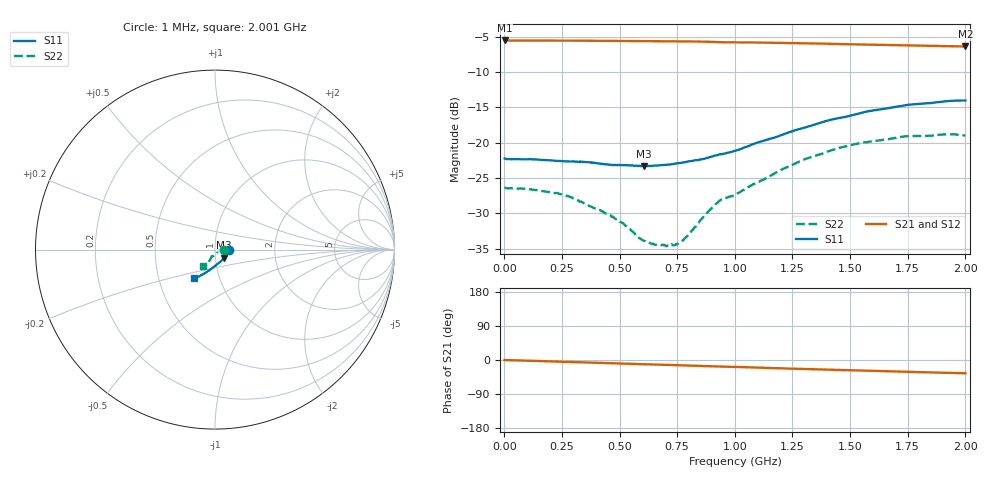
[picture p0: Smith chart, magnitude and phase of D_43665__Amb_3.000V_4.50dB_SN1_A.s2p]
! device id: 43665_
! dir: \\malibu\benchdata\1_engineers\tn_data\43665_75ohm\new\sparar\43665_\amb\3p000v\4p50db
! Serial: 1
! Insertion: A
! Temp: Amb
! VDD: 3.000V
! Attenuation Step: 4.50dB
! IDD: 1.453503e+00mA
! FILE NAME
! DATE 03-27-2009 08:34:29
! CORRECTED  DATA
#  Hz  S  RI  R  75
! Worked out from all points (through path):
!   401 points, 1 MHz to 2.001 GHz, reference 75 ohm
!   highest |S21| = -5.54 dB at 1 MHz (marker M1); lowest = -6.4 dB at 2.001 GHz (marker M2)
!   group delay of S21, straight-line fit = 49.6 ps
!   lowest |S11| = -23.3 dB at 606 MHz (marker M3), VSWR 1.15, Z = 82.6 - j7.57 ohm
!   |S11| at or under -10 dB: start of sweep to end of sweep
!   |S22| runs from -34.7 to -18.8 dB; largest |S21 - S12| = 0.0023
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1000000  0.0772 -0.00129  0.5282 -0.000748  0.5283 -0.000778  0.0484 -0.000475
1.06e8  0.0758 -0.00633  0.5271 -0.0173  0.5273 -0.0174  0.0469 0.00152
2.36e8  0.0727 -0.0149  0.5255 -0.0385  0.5257 -0.0387  0.0434 0.00178
3.36e8  0.0698 -0.0225  0.5234 -0.055  0.5236 -0.0552  0.0379 0.00188
4.81e8  0.0607 -0.0337  0.5191 -0.0791  0.5193 -0.0793  0.0288 -0.00283
6.06e8  0.0507 -0.0456  0.5137 -0.0993  0.5137 -0.0995  0.0184 -0.00823
6.71e8  0.0451 -0.0524  0.5108 -0.1101  0.5108 -0.1103  0.0141 -0.0125
7.11e8  0.041 -0.0565  0.5086 -0.1168  0.5086 -0.1168  0.0112 -0.015
7.41e8  0.0378 -0.0601  0.5069 -0.1219  0.5071 -0.1219  0.0086 -0.0167
7.61e8  0.0359 -0.0622  0.5057 -0.1252  0.5057 -0.1252  0.00669 -0.0185
7.96e8  0.032 -0.066  0.5034 -0.1311  0.5033 -0.1311  0.00349 -0.0216
8.66e8  0.0223 -0.0732  0.4979 -0.1429  0.4978 -0.1428  -0.00258 -0.0301
9.26e8  0.0137 -0.0806  0.4915 -0.1519  0.4918 -0.1516  -0.00969 -0.0364
9.46e8  0.0115 -0.0821  0.4895 -0.154  0.4898 -0.1538  -0.0132 -0.0373
1.001e9  0.00499 -0.0872  0.4866 -0.1601  0.4868 -0.1601  -0.0191 -0.0381
1.211e9  -0.0266 -0.1111  0.4703 -0.1916  0.4709 -0.1917  -0.0287 -0.0587
1.336e9  -0.0457 -0.1244  0.4581 -0.2076  0.4588 -0.208  -0.0366 -0.0705
1.511e9  -0.0716 -0.1393  0.4401 -0.2284  0.4406 -0.2294  -0.0467 -0.0847
1.671e9  -0.0914 -0.1502  0.4242 -0.2455  0.4238 -0.2466  -0.0542 -0.0913
1.741e9  -0.0995 -0.1545  0.417 -0.2522  0.4168 -0.2537  -0.0575 -0.0946
1.911e9  -0.1138 -0.1592  0.4005 -0.2673  0.3997 -0.2676  -0.0653 -0.0938
2.001e9  -0.1181 -0.1595  0.3922 -0.2747  0.3901 -0.2759  -0.0669 -0.09
